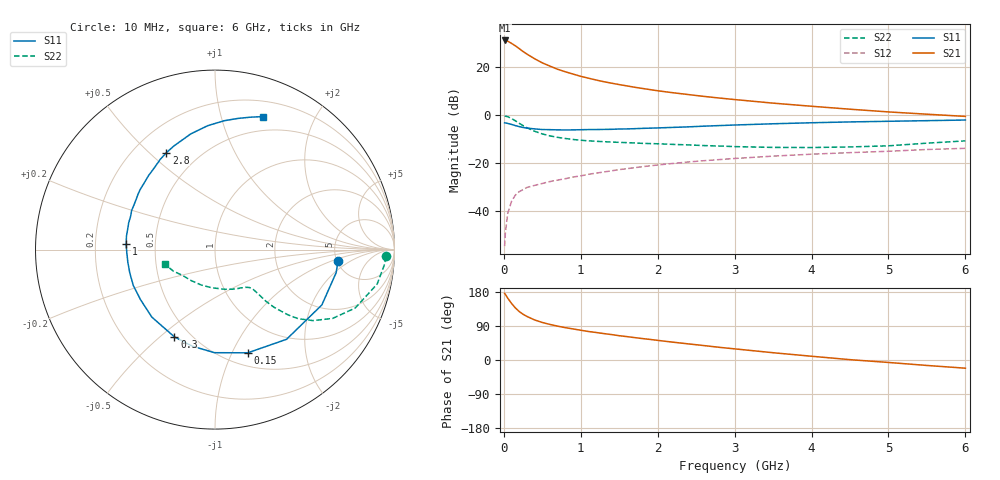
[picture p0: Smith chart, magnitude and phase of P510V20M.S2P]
! SIEMENS Small Signal Semiconductors
! BFP183
! Si NPN RF Bipolar Junction Transistor in SOT143
! VCE = 10 V  IC = 20 mA
! Common Emitter S-Parameters:  March  1996
# GHz  S  MA  R  50
!  f  S11  S21  S12  S22
! GHz  MAG  ANG  MAG  ANG  MAG  ANG  MAG  ANG
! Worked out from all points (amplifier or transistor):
!   36 points, 10 MHz to 6 GHz, reference 50 ohm
!   highest |S21| = 31.0 dB at 10 MHz (marker M1)
!   |S21| within 3 dB of that: start of sweep to 183.3 MHz
!   unconditionally stable (mu >= 1): 972.6 MHz to 5.886 GHz
!   at 250 MHz: K = 0.43, MSG = 28.7 dB, |S12| = -30.9 dB
!   at 1.4 GHz: K = 1.10, MAG = 16.3 dB, |S12| = -23.1 dB
!   at 6 GHz: K = 0.99, MSG = 6.6 dB, |S12| = -13.8 dB
!   S11 on the Smith chart (normalised r, x): 10 MHz: 5.12, -1.22; 150 MHz: 0.64, -1.15; 300 MHz: 0.41, -0.56; 1 GHz: 0.34, +0.03; 2.8 GHz: 0.33, +0.57; 6 GHz: 0.35, +1.37
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0.01  0.6886 -5.2  35.3 175.8  0.0019 73.0  0.9533 -2.3
0.02  0.6871 -10.8  35.1 173.1  0.0036 76.7  0.9489 -4.8
0.05  0.6704 -27.4  34.13 163.4  0.009 77.7  0.9236 -12.0
0.1  0.6393 -51.4  30.73 149.3  0.0162 64.6  0.8465 -22.6
0.15  0.6034 -72.4  27.27 137.4  0.0218 58.4  0.7597 -30.3
0.2  0.5744 -90.3  23.92 127.9  0.0257 55.2  0.6746 -35.9
0.25  0.5526 -103.4  20.81 120.7  0.0284 51.5  0.603 -39.7
0.3  0.5364 -114.9  18.42 115.0  0.0314 49.6  0.5456 -41.8
0.4  0.5151 -133.1  14.73 105.7  0.0347 48.0  0.461 -44.3
0.5  0.4999 -146.2  12.1 99.0  0.038 47.1  0.4058 -45.4
0.6  0.4972 -156.3  10.35 93.8  0.0417 47.4  0.3693 -45.6
0.7  0.4922 -164.7  8.897 89.3  0.0447 48.2  0.3442 -45.7
0.8  0.4906 -171.7  7.901 85.3  0.0478 48.9  0.326 -45.9
1  0.4959 176.5  6.362 78.5  0.0546 49.7  0.2999 -46.5
1.1  0.499 171.4  5.818 75.2  0.059 49.8  0.2916 -47.2
1.5  0.5132 154.9  4.285 64.1  0.0736 49.4  0.2711 -50.8
2.2  0.5542 131.9  2.901 47.0  0.099 45.7  0.2458 -62.6
2.8  0.604 116.6  2.255 33.5  0.1189 40.7  0.2275 -76.3
3.5  0.6588 101.8  1.766 19.2  0.1404 34.9  0.213 -95.7
4.5  0.7199 85.9  1.321 0.9  0.1659 26.1  0.2178 -127.6
5.5  0.7642 74.9  1.041 -14.4  0.1927 18.8  0.261 -152.6
6  0.7881 70.1  0.937 -21.6  0.2039 14.4  0.2911 -163.6
